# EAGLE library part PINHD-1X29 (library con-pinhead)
PIN HEADER
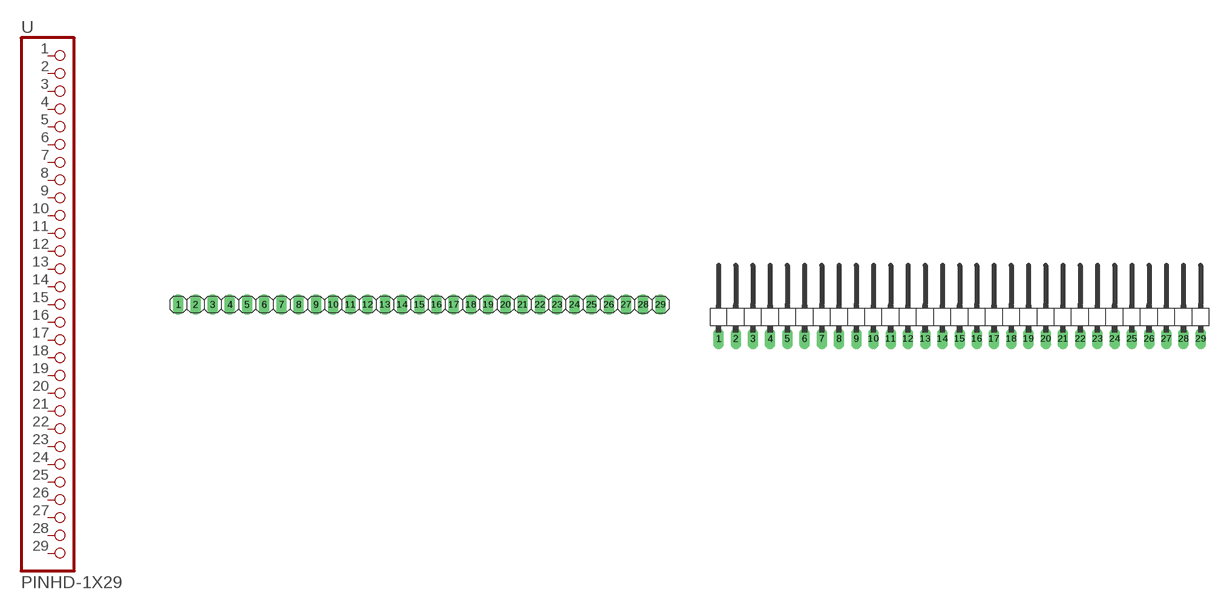
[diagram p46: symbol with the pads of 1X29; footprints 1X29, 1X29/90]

Designator prefix -

## PINHD-1X29_2.54  [1X29]
1  1  pas
2  2  pas
3  3  pas
4  4  pas
5  5  pas
6  6  pas
7  7  pas
8  8  pas
9  9  pas
10  10  pas
11  11  pas
12  12  pas
13  13  pas
14  14  pas
15  15  pas
16  16  pas
17  17  pas
18  18  pas
19  19  pas
20  20  pas
21  21  pas
22  22  pas
23  23  pas
24  24  pas
25  25  pas
26  26  pas
27  27  pas
28  28  pas
29  29  pas

## PINHD-1X29_2.54-90°  [1X29/90]
Pads as for 1X29

## PINHD-1X29_2.00  [1X29M]
Pads as for 1X29

## PINHD-1X29_2.54-SMD  [1X29SMD]
Pads as for 1X29

## PINHD-1X29_2.54-SMD-90°  [1X29SMD/90]
Pads as for 1X29

## Footprint 1X29 (pad centres in mm)
PIN HEADER - 2.54
drill 1.016 long: 1 -29.21,0; 2 -26.67,0; 3 -24.13,0; 4 -21.59,0; 5 -19.05,0; 6 -16.51,0; 7 -13.97,0; 8 -11.43,0; 9 -8.89,0; 10 -6.35,0; 11 -3.81,0; 12 -1.27,0; 13 1.27,0; 14 3.81,0; 15 6.35,0; 16 8.89,0; 17 11.43,0; 18 13.97,0; 19 16.51,0; 20 19.05,0; 21 21.59,0; 22 24.13,0; 23 26.67,0; 24 29.21,0; 25 31.75,0; 26 34.29,0; 27 36.83,0; 28 39.37,0; 29 41.91,0

## Footprint 1X29/90 (pad centres in mm)
PIN HEADER - 2.54 90°
drill 1.016 long: 1 -24.13,-3.81; 2 -21.59,-3.81; 3 -19.05,-3.81; 4 -16.51,-3.81; 5 -13.97,-3.81; 6 -11.43,-3.81; 7 -8.89,-3.81; 8 -6.35,-3.81; 9 -3.81,-3.81; 10 -1.27,-3.81; 11 1.27,-3.81; 12 3.81,-3.81; 13 6.35,-3.81; 14 8.89,-3.81; 15 11.43,-3.81; 16 13.97,-3.81; 17 16.51,-3.81; 18 19.05,-3.81; 19 21.59,-3.81; 20 24.13,-3.81; 21 26.67,-3.81; 22 29.21,-3.81; 23 31.75,-3.81; 24 34.29,-3.81; 25 36.83,-3.81; 26 39.37,-3.81; 27 41.91,-3.81; 28 44.45,-3.81; 29 46.99,-3.81

## Footprint 1X29M (pad centres in mm)
PIN HEADER - 2
drill 0.914 square: 1 -24,0
drill 0.914: 2 -22,0; 3 -20,0; 4 -18,0; 5 -16,0; 6 -14,0; 7 -12,0; 8 -10,0; 9 -8,0; 10 -6,0; 11 -4,0; 12 -2,0; 13 0,0; 14 2,0; 15 4,0; 16 6,0; 17 8,0; 18 10,0; 19 12,0; 20 14,0; 21 16,0; 22 18,0; 23 20,0; 24 22,0; 25 24,0; 26 26,0; 27 28,0; 28 30,0; 29 32,0

## Footprint 1X29SMD (pad centres in mm)
PIN HEADER - 2.54 SMD
smd 1.016 x 3.302: 1 -1.27,1.27; 2 1.27,-1.27; 3 3.81,1.27; 4 6.35,-1.27; 5 8.89,1.27; 6 11.43,-1.27; 7 13.97,1.27; 8 16.51,-1.27; 9 19.05,1.27; 10 21.59,-1.27; 11 24.13,1.27; 12 26.67,-1.27; 13 29.21,1.27; 14 31.75,-1.27; 15 34.29,1.27; 16 36.83,-1.27; 17 39.37,1.27; 18 41.91,-1.27; 19 44.45,1.27; 20 46.99,-1.27; 21 49.53,1.27; 22 52.07,-1.27; 23 54.61,1.27; 24 57.15,-1.27; 25 59.69,1.27; 26 62.23,-1.27; 27 64.77,1.27; 28 67.31,-1.27; 29 69.85,1.27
